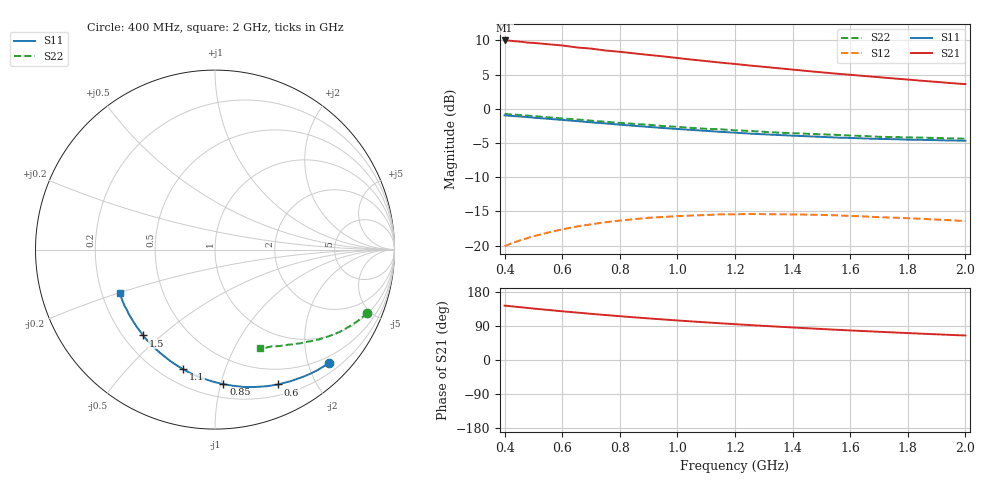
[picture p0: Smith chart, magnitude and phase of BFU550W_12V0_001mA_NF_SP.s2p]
! Filename:  P:\Prog\Test\Noise\ATS_data\Testdata_Net\06 Compressed Noise after Statistics\BFU550W_APM2013_11_D05_12p0V_001mA_NF_CM01_D.sf
! Date/Time: Tue 26/Mar/2013 16:25:24
! BFU550W_APM2013_11_D05_12p0V_1to35mA_NF_CM01_Bias1_R.sf
! Noise Parameter Data File
! BFU550W_APM2013_11_D05_12p0V_1to35mA_NF_CM01
! Date/time: Mon Mar 25 15:58:35 2013
! freq range =  0.4000 to  2.0000 GHz, 37 points
! bias range =  0.9950 to 34.9900 mA, 9 points
! bias supplies used: 1 1 0 0 0 0
! VAR bias_mode= 1  ! Specify V_out, I_out
! VAR bias_var = 1  ! Bias variable = I_out
! VAR V_out= 12.001000
! VAR I_out= 0.995000
! VAR V_in= 0.771500
! VAR I_in= 0.007500
! Device data file deembeded for feedlines and parallel
! Original file: \06 Compressed Noise after Statistics\BFU550W_APM2013_11_D05_12p0V_001mA_NF_CM01_R.sf
! Feed-files: PR019V01_070313_Feed1.s2p, PR019V01_070313_Feed2.s2p
! Parallel-file: PR019V01_070313_Par.s2p
# MHz S MA R 50
!  Freq-MHz  S11-mag  S11-arg  S21-mag  S21-arg  S12-mag  S12-arg  S22-mag  S22-arg
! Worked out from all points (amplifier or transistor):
!   37 points, 400 MHz to 2 GHz, reference 50 ohm
!   highest |S21| = 10.0 dB at 400 MHz (marker M1)
!   |S21| within 3 dB of that: start of sweep to 1.096 GHz
!   unconditionally stable (mu >= 1): nowhere
!   at 500 MHz: K = 0.20, MSG = 14.1 dB, |S12| = -18.6 dB
!   at 1.1 GHz: K = 0.42, MSG = 11.3 dB, |S12| = -15.5 dB
!   at 2 GHz: K = 0.80, MSG = 10.0 dB, |S12| = -16.4 dB
!   lowest NFmin = 0.48 dB at 420 MHz
!   S11 on the Smith chart (normalised r, x): 400 MHz: 0.37, -2.37; 600 MHz: 0.32, -1.53; 850 MHz: 0.30, -1.02; 1.1 GHz: 0.29, -0.73; 1.5 GHz: 0.28, -0.44; 2 GHz: 0.27, -0.20
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400  0.896 -45.0  3.16 143.7  0.09912 62.0  0.9171 -22.5
420  0.8891 -47.1  3.145 142.0  0.1031 60.8  0.9114 -23.4
440  0.8829 -49.1  3.116 140.4  0.1068 59.6  0.9056 -24.4
480  0.8696 -53.1  3.049 137.4  0.1137 57.3  0.8919 -26.2
500  0.8624 -55.2  3.034 135.8  0.117 56.2  0.8851 -27.1
600  0.8297 -64.9  2.906 128.6  0.1315 51.0  0.8508 -31.1
650  0.814 -69.3  2.81 125.2  0.1379 48.8  0.836 -32.9
700  0.7966 -73.9  2.756 121.8  0.1432 46.5  0.8191 -34.9
750  0.7822 -78.1  2.669 118.7  0.1482 44.4  0.8046 -36.4
800  0.7657 -82.3  2.611 115.6  0.1524 42.4  0.7895 -38.1
850  0.7511 -86.5  2.542 112.6  0.1562 40.5  0.7756 -39.6
950  0.7242 -94.2  2.418 107.0  0.1619 37.1  0.7487 -42.5
1000  0.7122 -98.0  2.352 104.3  0.1645 35.5  0.7383 -43.7
1100  0.6896 -105.0  2.232 99.3  0.1674 32.8  0.7145 -46.4
1200  0.6694 -111.7  2.127 94.5  0.1694 30.4  0.6961 -48.8
1250  0.6594 -115.0  2.074 92.2  0.1704 29.2  0.6893 -49.7
1350  0.6441 -121.2  1.981 87.9  0.1695 27.4  0.6702 -52.1
1500  0.6236 -129.9  1.85 81.8  0.1678 25.1  0.6511 -55.4
1600  0.6128 -135.5  1.773 78.0  0.1648 24.2  0.638 -57.6
1750  0.5999 -143.2  1.668 72.8  0.1603 23.6  0.622 -60.5
1850  0.5933 -148.2  1.603 69.4  0.157 23.4  0.616 -62.5
2000  0.5852 -155.3  1.516 64.6  0.1513 24.3  0.604 -65.6
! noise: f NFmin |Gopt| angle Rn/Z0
400  0.4902  0.6701  30.25  0.3059
460  0.5126  0.6651  35.68  0.3261
600  0.5842  0.6709  42.74  0.3307
800  0.653  0.6407  57.94  0.2753
1000  0.8204  0.638  71.25  0.2926
1200  0.8898  0.6222  86.53  0.2345
1400  0.8725  0.6261  101  0.1854
1600  0.7647  0.604  115.5  0.1321
1800  1.024  0.6177  128.8  0.1159
2000  1.12  0.6505  140.2  0.0868
